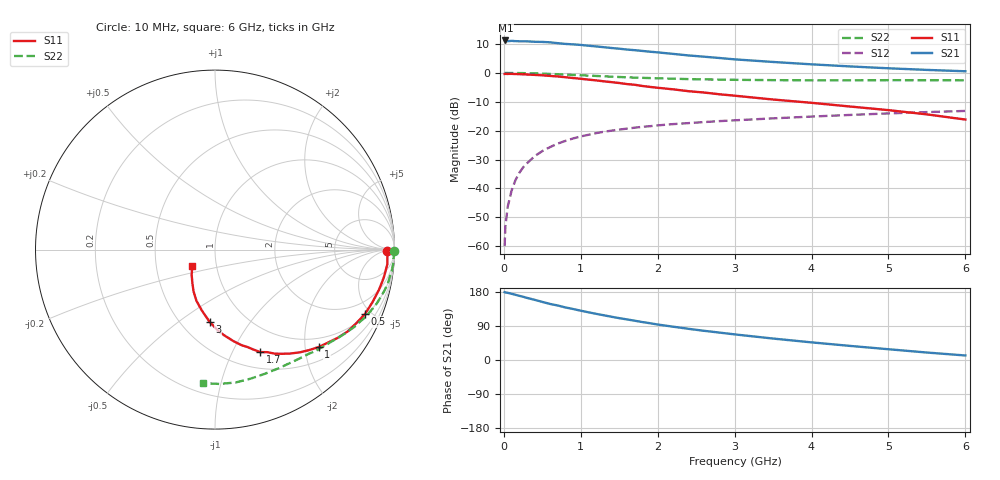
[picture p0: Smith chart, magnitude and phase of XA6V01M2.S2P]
! SIEMENS Discrete & RF Semiconductors
! BFY180
! Si NPN RF Bipolar Junction Transistor in MICRO-X
! VCE = 6 V  IC = 1.2 mA
! Common Emitter S-Parameters:  May  1997
# GHz  S  MA  R  50
!  f  S11  S21  S12  S22
! GHz  MAG  ANG  MAG  ANG  MAG  ANG  MAG  ANG
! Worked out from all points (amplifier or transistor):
!   36 points, 10 MHz to 6 GHz, reference 50 ohm
!   highest |S21| = 11.2 dB at 20 MHz (marker M1)
!   |S21| within 3 dB of that: start of sweep to 1.55 GHz
!   unconditionally stable (mu >= 1): 3.813 GHz to end of sweep
!   at 250 MHz: K = 0.09, MSG = 21.8 dB, |S12| = -32.7 dB
!   at 1.4 GHz: K = 0.53, MSG = 14.3 dB, |S12| = -20.0 dB
!   at 6 GHz: K = 1.06, MAG = 5.4 dB, |S12| = -13.2 dB
!   S11 on the Smith chart (normalised r, x): 10 MHz: 48, -8; 500 MHz: 1.11, -4.61; 1 GHz: 0.78, -2.29; 1.7 GHz: 0.69, -1.29; 3 GHz: 0.68, -0.66; 6 GHz: 0.76, -0.14
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0.01  0.9603 -0.4  3.599 179.0  0.001 83.3  0.9968 -0.3
0.02  0.9624 -0.9  3.65 178.4  0.0022 93.3  0.9999 -0.6
0.05  0.9611 -2.2  3.542 177.3  0.0048 85.6  0.9974 -1.4
0.1  0.9639 -4.7  3.592 174.8  0.0091 90.4  0.9956 -2.8
0.15  0.9575 -7.3  3.554 172.1  0.0138 85.7  0.9967 -4.2
0.25  0.9462 -11.7  3.535 166.9  0.0231 82.2  0.9928 -7.0
0.5  0.9095 -23.2  3.444 153.3  0.0443 74.3  0.9718 -13.5
0.6  0.8874 -27.6  3.387 147.9  0.0519 71.3  0.9603 -16.0
0.8  0.8423 -35.7  3.18 138.7  0.0665 65.7  0.9362 -20.8
1  0.7924 -43.3  3.053 130.1  0.0795 60.4  0.9117 -25.1
1.1  0.7662 -47.0  2.959 125.9  0.0849 58.5  0.8978 -27.1
1.4  0.6922 -57.0  2.702 114.1  0.1001 52.2  0.8614 -32.9
1.7  0.624 -66.2  2.478 103.7  0.1126 47.5  0.8295 -37.8
2  0.5532 -74.4  2.268 93.6  0.1235 43.5  0.8072 -42.3
2.2  0.5202 -78.6  2.137 87.9  0.1299 40.9  0.7954 -45.3
2.6  0.4581 -87.1  1.912 77.1  0.1408 36.9  0.773 -50.5
3  0.4036 -94.3  1.719 67.6  0.1511 33.2  0.7594 -55.6
3.5  0.3464 -102.3  1.548 56.6  0.1634 29.5  0.7503 -61.7
4  0.3037 -109.9  1.409 46.5  0.1755 25.7  0.7457 -68.0
4.5  0.2621 -117.1  1.296 37.2  0.1873 21.9  0.7459 -74.5
5.5  0.1914 -132.8  1.128 19.7  0.2098 14.3  0.7488 -88.2
6  0.1558 -144.4  1.068 11.9  0.2197 10.0  0.7465 -95.1
